(* Logix 5000 AddOnInstructionDefinition export CFW900_120170; software revision 20.06 *)

ADD_ON_INSTRUCTION CFW900_120170   (* revision 1.0, ExecutePrescan *)
// 120/170 CIP Basic Speed
// AOI plus parameters
// Help:
// Drive setup as follows:
// C9.5.1 = 120/170
// C9.5.2 = 1
// C9.5.3 = 8
// C9.5.4 = 1
// C9.5.5 = 8
// C9.2.1.1 - 3
// C9.2.1.2 - 7
// C9.2.1.3 - 5
// C9.2.1.4 - 60
// C9.2.1.5 - USER DEFINED
// C9.2.1.6 - USER DEFINED
// C9.2.1.7 - USER DEFINED
// C9.2.1.8 - USER DEFINED
// C9.2.2.2 - 100
// C9.2.2.3 - 101
// C9.2.2.4 - USER DEFINED
// C9.2.2.5 - USER DEFINED
// C9.2.2.6 - USER DEFINED
// C9.2.2.7 - USER DEFINED
// C9.2.2.8- USER DEFINED
// C4.1.1 - Remote 2
// C4.2.2.1 - Ethernet
// C4.2.2.2 - Ethernet
// C4.2.2.3 - Ethernet
// C4.2.2.4 - Ethernet
// C4.3.1.2.1 - Keypad
// C4.3.1.2.2 - Ethernet
VAR_INPUT
   ConnectionFaulted : BOOL; {required}   // From CFW900
END_VAR
VAR_IN_OUT
   Inputs : INT[10]; {required}   // Input Assembly From CFW900
   Outputs : INT[10]; {required}   // Output Assembly To CFW900
END_VAR
VAR_INPUT
   Run : BOOL; {visible}   // 1 = Run 0 = Stop
   Fault_Reset : BOOL; {visible}   // 1 = Clear fault 0 = no action
   cfg_FailToStartDelay : DINT; {visible}   // Time in seconds before faulting on fail to start if vfd doesn't start on command (0 to disable)
   cfg_FailToStopDelay : DINT; {visible}   // Time in seconds before faulting on fail to stop if vfd doesn't stop on command (0 to disable)
END_VAR
VAR_OUTPUT
   Connection_Ready : BOOL; {access Read Only, visible}   // 1 = Connection to VFD is established to PLC
   Connection_Faulted : BOOL; {access Read Only, visible}   // Connection_Faulted Status Bit
   Running : BOOL; {access Read Only, visible}   // 1 = CFW900 Running 0 = CFW900 Stopped
   Faulted : BOOL; {access Read Only, visible}   // AOI Faulted Connection fault or failed to start / stop as well as VFD faults
END_VAR
VAR_INPUT
   Speed_Reference : INT; {required}   // Speed Setpoint (RPM) Negative speed will reverse direction
END_VAR
VAR_OUTPUT
   RealSpeed : INT; {access Read Only, visible}   // Current Speed (RPM)
   val_OutputCurrent : REAL; {access Read Only, visible}
   val_OutputVoltage : REAL; {access Read Only, visible}
   val_OutputFreq : REAL; {access Read Only, visible}
   val_FaultCode : DINT; {access Read Only, visible}
END_VAR
VAR_INPUT
   set_Accel : REAL := 10.0; {required}   // Acceleration Ramp setpoint (0.1-999.9) in seconds
   set_Decel : REAL := 10.0; {required}   // Deceleration Ramp setpoint (0.1-999.9) in seconds
END_VAR
VAR
   FailToStart : TIMER; {access None}
   FailToStop : TIMER;
   Wrk_Run1 : BOOL; {access None}
   TempReal : REAL; {access None}
   TempDINT : DINT; {access None}
END_VAR

ROUTINE Logic   (* ladder *)
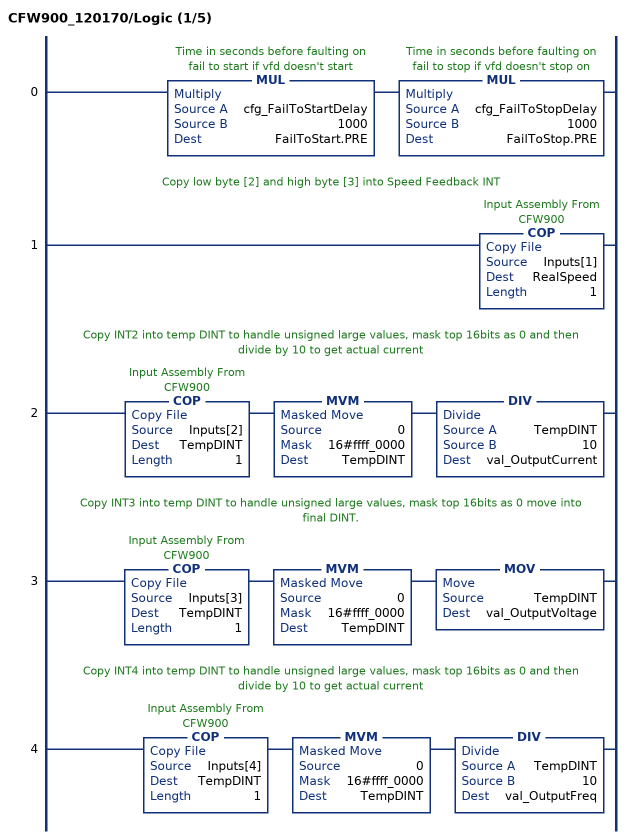
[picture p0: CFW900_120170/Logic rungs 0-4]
   0: MUL(cfg_FailToStartDelay,1000,FailToStart.PRE)MUL(cfg_FailToStopDelay,1000,FailToStop.PRE);
   // Copy low byte [2] and high byte [3] into Speed Feedback INT
   1: COP(Inputs[1],RealSpeed,1);
   // Copy INT2 into temp DINT to handle unsigned large values, mask top 16bits as 0 and then divide by 10 to get actual current
   2: COP(Inputs[2],TempDINT,1)MVM(0,16#ffff_0000,TempDINT)DIV(TempDINT,10,val_OutputCurrent);
   // Copy INT3 into temp DINT to handle unsigned large values, mask top 16bits as 0 move into final DINT.
   3: COP(Inputs[3],TempDINT,1)MVM(0,16#ffff_0000,TempDINT)MOV(TempDINT,val_OutputVoltage);
   // Copy INT4 into temp DINT to handle unsigned large values, mask top 16bits as 0 and then divide by 10 to get actual current
   4: COP(Inputs[4],TempDINT,1)MVM(0,16#ffff_0000,TempDINT)DIV(TempDINT,10,val_OutputFreq);
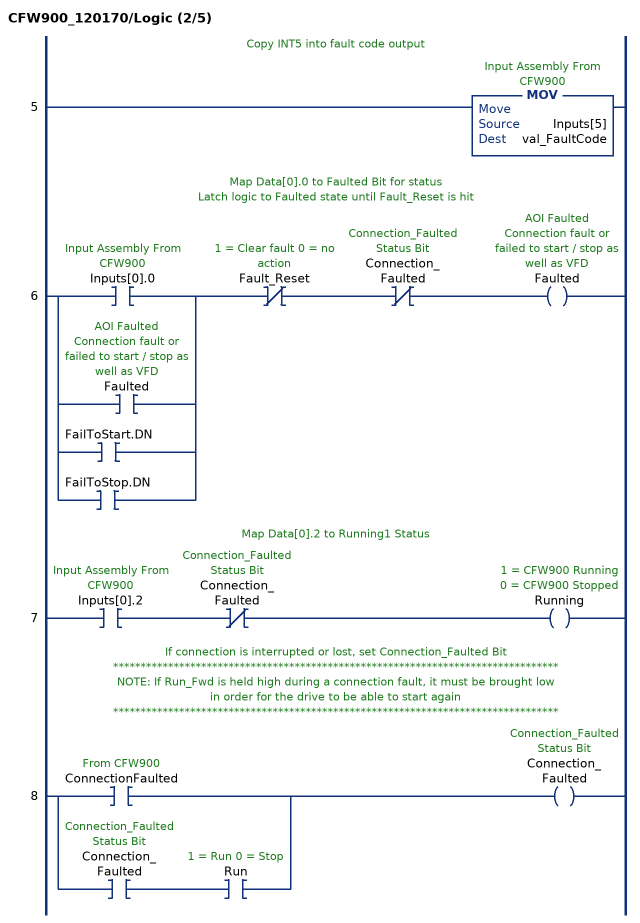
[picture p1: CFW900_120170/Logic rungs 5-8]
   // Copy INT5 into fault code output
   5: MOV(Inputs[5],val_FaultCode);
   // Map Data[0].0 to Faulted Bit for status
   // Latch logic to Faulted state until Fault_Reset is hit
   6: [XIC(Inputs[0].0) ,XIC(Faulted) ,XIC(FailToStart.DN) ,XIC(FailToStop.DN) ]XIO(Fault_Reset)XIO(Connection_Faulted)OTE(Faulted);
   // Map Data[0].2 to Running1 Status
   7: XIC(Inputs[0].2)XIO(Connection_Faulted)OTE(Running);
   // If connection is interrupted or lost, set Connection_Faulted Bit
   // *********************************************************************************
   // NOTE: If Run_Fwd is held high during a connection fault, it must be brought low
   // in order for the drive to be able to start again
   // *********************************************************************************
   8: [XIC(ConnectionFaulted) ,XIC(Connection_Faulted) XIC(Run) ]OTE(Connection_Faulted);
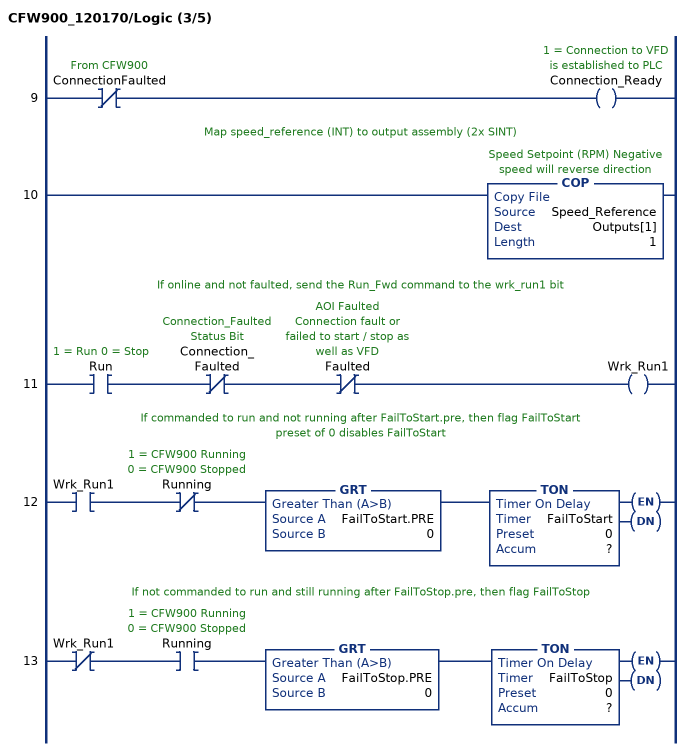
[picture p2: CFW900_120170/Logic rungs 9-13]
   9: XIO(ConnectionFaulted)OTE(Connection_Ready);
   // Map speed_reference (INT) to output assembly (2x SINT)
   10: COP(Speed_Reference,Outputs[1],1);
   // If online and not faulted, send the Run_Fwd command to the wrk_run1 bit
   11: XIC(Run)XIO(Connection_Faulted)XIO(Faulted)OTE(Wrk_Run1);
   // If commanded to run and not running after FailToStart.pre, then flag FailToStart
   // preset of 0 disables FailToStart
   12: XIC(Wrk_Run1)XIO(Running)GRT(FailToStart.PRE,0)TON(FailToStart,?,?);
   // If not commanded to run and still running after FailToStop.pre, then flag FailToStop
   13: XIO(Wrk_Run1)XIC(Running)GRT(FailToStop.PRE,0)TON(FailToStop,?,?);
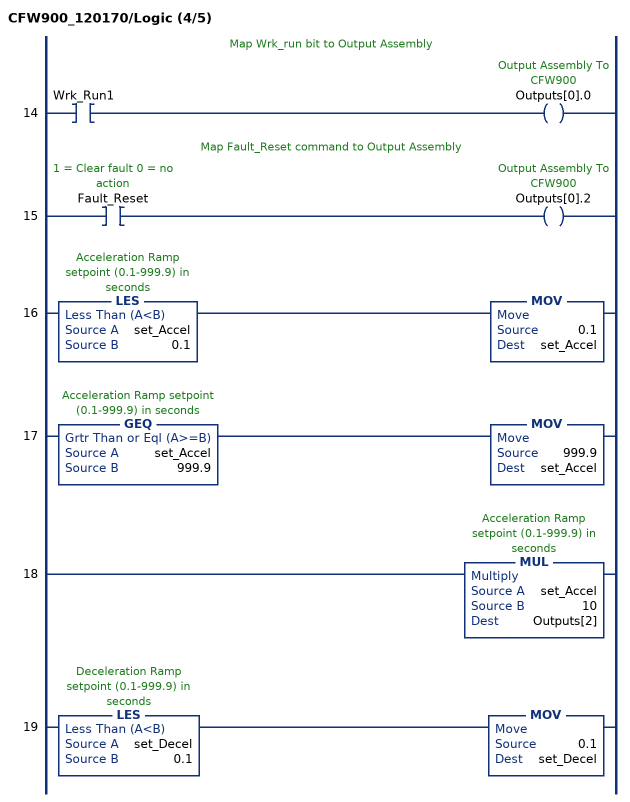
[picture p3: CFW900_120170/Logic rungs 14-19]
   // Map Wrk_run bit to Output Assembly
   14: XIC(Wrk_Run1)OTE(Outputs[0].0);
   // Map Fault_Reset command to Output Assembly
   15: XIC(Fault_Reset)OTE(Outputs[0].2);
   16: LES(set_Accel,0.1)MOV(0.1,set_Accel);
   17: GEQ(set_Accel,999.9)MOV(999.9,set_Accel);
   18: MUL(set_Accel,10,Outputs[2]);
   19: LES(set_Decel,0.1)MOV(0.1,set_Decel);
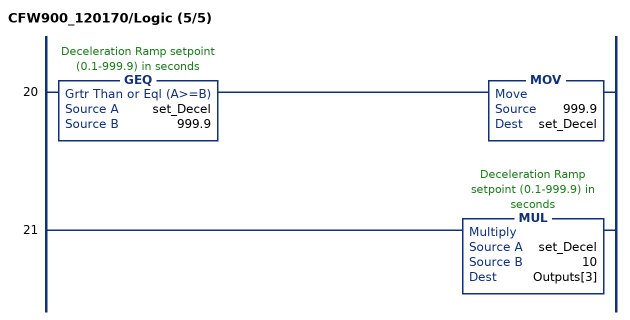
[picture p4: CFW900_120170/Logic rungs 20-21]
   20: GEQ(set_Decel,999.9)MOV(999.9,set_Decel);
   21: MUL(set_Decel,10,Outputs[3]);
END_ROUTINE

ROUTINE Prescan   (* ladder *)
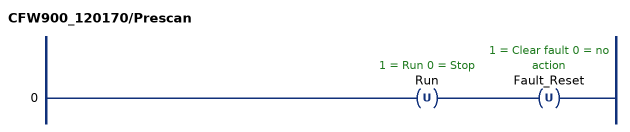
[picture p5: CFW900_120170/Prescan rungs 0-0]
   0: OTU(Run)OTU(Fault_Reset);
END_ROUTINE
END_ADD_ON_INSTRUCTION
